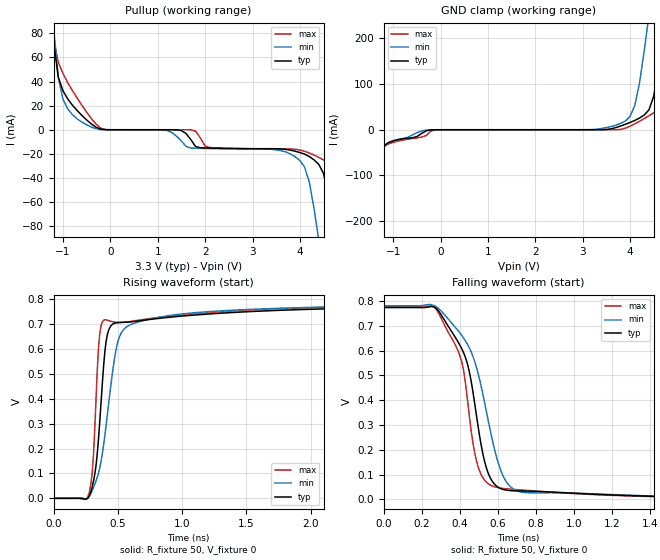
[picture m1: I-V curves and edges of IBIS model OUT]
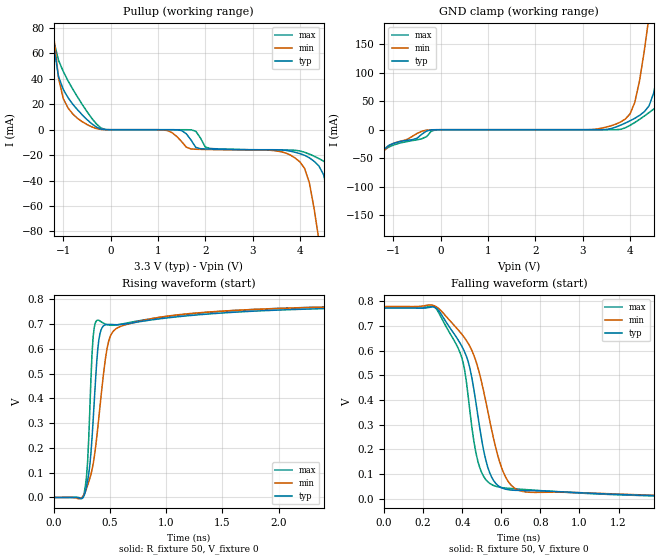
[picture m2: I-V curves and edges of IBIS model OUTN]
|   IBIS File of SG2520HGN C
|   HCSL Zdiff=100, Vcc=3.3V, fo<=212.5MHz
[IBIS Ver]   3.2
[File Name]   sg2520hgn_33v.ibs
[File Rev]   1.0
[Date]   Jan. 25, 2023
[Source]
[Notes]
Created by Minoru Kozaki
[Disclaimer]
Seiko Epson Corporation makes no warranty with respect to the
information contained herein.
[Copyright]
Copyright(C) 2023, Seiko Epson Corporation. All rights reserved.
|   Component
[Component]   SG2520HGN
[Manufacturer]  Seiko Epson Corporation
[Package]
R_pkg   17.7m   NA   NA
L_pkg   235p   NA   NA
C_pkg   208f   NA   NA
[Pin]   signal_name   model_name   R_pin   L_pin   C_pin
1   OE/ST   NC
2   NC   NC
3   GND   GND
4   OUT   OUT   17.7m   235p   208f
5   OUTN   OUTN   10.4m   129p   221f
6   VCC   POWER
[Diff Pin] inv_pin  vdiff  tdelay_typ
4   5   0   0
| Models and submodels in the file (2): OUT (Open_source), OUTN (Open_source)
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|   Model OUT
[Model]   OUT
Model_type   Open_source
Polarity   Non-Inverting
Vref = 0
Vmeas = 0.4
Rref = 50
Cref = 0
C_comp   12.0p   12.0p   12.0p
[Temperature Range]   25   105   -40
[Voltage Range]   3.3   2.97   3.63
[Pullup Reference]   3.3   2.97   3.63
[GND Clamp Reference]   0   0   0
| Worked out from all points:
|   GND clamp passes 1 mA (typ) near -0.23 V on its own axis
|   falling waveform, R_fixture 50, V_fixture 0: 20-80 % time 127ps typ, 157ps min, 111ps max; typ from 0.773 V to 0 V
|   rising waveform, R_fixture 50, V_fixture 0: 20-80 % time 70.9ps typ, 125ps min, 44.5ps max; typ from 0 V to 0.772 V
[Pullup]
-3.3V     2.127A     2.05A      2.21A
-1.3V     132.8mA    150.2mA    126.6mA
-1.2V     73.45mA    84.87mA    75.8mA
-1.1V     43.67mA    43.61mA    56mA
-1V       32.23mA    25.14mA    46.62mA
-200mV    439uA      190.2uA    1.261mA
3.8V      -16.94mA   -20.08mA   -15.98mA
4.1V      -20.27mA   -31.07mA   -17.88mA
4.4V      -28.81mA   -91.77mA   -22.96mA
4.8V      -110.1mA   -195.7mA   -36.13mA
5.1V      -195.3mA   -273.8mA   -103.4mA
6.6V      -622.1mA   -665.7mA   -565.9mA
[GND Clamp]
-3.3V     -621.5mA   -578.2mA   -668.1mA
-1.9V     -222.4mA   -213.1mA   -234.4mA
-1.3V     -53.21mA   -57.58mA   -52.09mA
-1V       -24.39mA   -24.08mA   -27.51mA
3.9V      11.83mA    19.11mA    3.407mA
4.1V      20.31mA    53.2mA     12.88mA
4.4V      43.67mA    251.8mA    30.61mA
4.5V      73.45mA    331mA      37.06mA
4.7V      212.7mA    491.1mA    52.8mA
4.8V      297.2mA    571.7mA    67.46mA
5.1V      556.7mA    815.8mA    267.3mA
6.6V      2.127A     2.436A     1.769A
[Falling Waveform]
R_fixture = 50
V_fixture = 0
V_fixture_min = 0
V_fixture_max = 0
0s        773.3mV    780.1mV    777.8mV
250ps     777.4mV    785mV      780.4mV
300ps     746.6mV    761.1mV    733.5mV
410ps     607.8mV    661.4mV    556mV
470ps     429.5mV    575.1mV    223.1mV
530ps     154.4mV    392.1mV    77.92mV
590ps     55.67mV    179.4mV    49.28mV
650ps     36.71mV    65.17mV    42.39mV
750ps     33.44mV    27.05mV    36.47mV
4ns       337uV      504uV      270uV
[Rising Waveform]
R_fixture = 50
V_fixture = 0
V_fixture_min = 0
V_fixture_max = 0
0s        123uV      178uV      112uV
270ps     2.257mV    4.33mV     9.849mV
300ps     44.44mV    30.16mV    98.92mV
330ps     130.1mV    69.61mV    392.5mV
360ps     312.1mV    123.2mV    663.3mV
390ps     535.2mV    216.4mV    715.9mV
430ps     677.6mV    386.4mV    713.9mV
500ps     706.2mV    628.5mV    706.3mV
650ps     712mV      707.4mV    714.7mV
4ns       772.2mV    778.7mV    777mV
[Ramp]
R_load = 50
dV/dt_r   0.47160/72.38p   0.47516/129.62p   0.47483/45.08p
dV/dt_f   0.47160/133.72p   0.47516/163.49p   0.47483/117.35p
|   Model OUTN
[Model]   OUTN
Model_type   Open_source
Polarity   Inverting
Vref = 0
Vmeas = 0.4
Rref = 50
Cref = 0
C_comp   12.0p   12.0p   12.0p
[Temperature Range]   25   105   -40
[Voltage Range]   3.3   2.97   3.63
[Pullup Reference]   3.3   2.97   3.63
[GND Clamp Reference]   0   0   0
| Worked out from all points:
|   GND clamp passes 1 mA (typ) near -0.23 V on its own axis
|   falling waveform, R_fixture 50, V_fixture 0: 20-80 % time 124ps typ, 154ps min, 107ps max; typ from 0.773 V to 0 V
|   rising waveform, R_fixture 50, V_fixture 0: 20-80 % time 70.6ps typ, 126ps min, 44ps max; typ from 0 V to 0.771 V
[Pullup]
-3.3V     1.49A      1.465A     1.529A
-1.3V     108.6mA    121.8mA    105.2mA
-1.2V     65.04mA    73.08mA    69.68mA
-1.1V     41.78mA    40.49mA    54.54mA
-900mV    25.24mA    17.07mA    38.41mA
-200mV    437.9uA    190uA      1.252mA
3.8V      -16.9mA    -20mA      -15.98mA
4.1V      -20.14mA   -30.53mA   -17.78mA
4.4V      -28.45mA   -86.52mA   -22.7mA
4.8V      -103.1mA   -184.6mA   -35.34mA
5.1V      -183mA     -258.2mA   -96.2mA
6.6V      -583.3mA   -627.8mA   -527.4mA
[GND Clamp]
-3.3V     -582.6mA   -545.3mA   -622.6mA
-1.8V     -181.8mA   -176.5mA   -189.6mA
-1.2V     -34.5mA    -37.04mA   -35.88mA
-200mV    -325.9uA   -114.8uA   -2.456mA
3.8V      8.003mA    13.65mA    676.4uA
4.1V      20.06mA    48.33mA    12.68mA
4.4V      41.78mA    199.4mA    30.1mA
4.5V      65.04mA    261.4mA    36.42mA
4.7V      166.7mA    386.3mA    51.67mA
4.8V      231.3mA    449.2mA    63.66mA
5.1V      429.8mA    638.8mA    205.8mA
6.6V      1.49A      1.741A     1.278A
[Falling Waveform]
R_fixture = 50
V_fixture = 0
V_fixture_min = 0
V_fixture_max = 0
0s        772.5mV    779.2mV    776.9mV
260ps     775.6mV    781.3mV    776.4mV
380ps     642.7mV    683.9mV    609.1mV
440ps     526.8mV    616.5mV    351.2mV
480ps     337.7mV    532.4mV    152.4mV
530ps     130.1mV    358.6mV    69.49mV
580ps     55.67mV    181.1mV    48.87mV
640ps     36.23mV    64.86mV    42.13mV
740ps     33.23mV    26.56mV    36.41mV
4ns       330uV      491uV      265uV
[Rising Waveform]
R_fixture = 50
V_fixture = 0
V_fixture_min = 0
V_fixture_max = 0
0s        113uV      180uV      111uV
270ps     8.091mV    12.57mV    17.37mV
300ps     66.09mV    48.21mV    139.1mV
350ps     312.5mV    135.4mV    649.6mV
390ps     594.1mV    276.7mV    716.1mV
420ps     676.4mV    407.8mV    709.9mV
490ps     698.8mV    634.2mV    696.3mV
620ps     699.4mV    695mV      701.8mV
1.6ns     747.9mV    755.2mV    754.8mV
4ns       771.2mV    777.5mV    776mV
[Ramp]
R_load = 50
dV/dt_r   0.47151/72.26p   0.47508/131.41p   0.47470/44.58p
dV/dt_f   0.47151/130.03p   0.47508/160.30p   0.47470/113.34p
